|Texas Instruments Incorporated
|8 Channel, SPI, Voltage-Output DAC With Precision Internal Reference
[IBIS Ver]   4.1
[File name]   dacx0508.ibs
[File Rev]   4.0
[Date]   06/21/2018
[Source]
| Texas Instruments Incorporated.
| 12500 TI Blvd
| Dallas, TX -75243
[Notes]   Revision History:
| Rev 4.1: 08/20/2021
| - Added SDO pin Hi-Z mode option version for DAC80508
| Rev 4.0: 06/21/2018
| - Added CLR version for DAC60508 and DAC80508
| Rev 3.0: 05/10/2018
| - Added model for 3.3V operation.
| - Updated C_comp values
| - Model generated from simulations in SPECTRE
| Rev 2.0: 01/17/2018
| - Added YZF package
| Rev 1.0: 01/27/2017
| - Initial version of the model
| - Model generated from simulations in TISPICE
| - C_comp although listed in numerical order of value are
|   obtained from varying PVT conditions. For PVT conditions for
|   each specific value refer the buffer description under
|   respective [Model]. IBIS model user is responsible for using
|   appropriate C_comp to simulate for Signal Integrity.
| - Warnings regarding combined Non-monotonicity of various models have been
|   reviewd and considered minor and can be ignored.
| - Model names with a trailing _1p8 contain the model for
|   1.8V operation. Model names with a trailing _3p0 contain the model
|   for 3.0V operation.Model names with a trailing _3p3 contain the model
|   for 3.3V operation.Model names with a trailing _5p0 contain the model
|   for 5.0V operation.
[Disclaimer]
| This model is designed as an aid for customers of Texas Instruments.
| TI and its licensors and suppliers make no warranties, either expressed
| or implied, with respect to this  model, including the warranties of
| merchantability or fitness for a particular purpose. The model is
| provided solely on an "as is" basis. The entire risk as to its quality
| and performance is with the customer.
| This model is subject to change without notice. Texas Instruments
| Incorporated is not responsible for updating this model.
[Copyright]
 (C) Copyright 2018 Texas Instruments Incorporated.All rights reserved.
| Component DAC60508MRTE
| 16 pin WQFN
| Part # DAC60508MRTE
[Component]   DAC60508MRTE
[Manufacturer]  TI
[Package]   |16 pin WQFN
| variable   typ   min   max
R_pkg   0.1   0.08   0.12
L_pkg   1.0nH   0.8nH   1.2nH
C_pkg   0.2pF   0.16pF   0.24pF
[Pin]  signal_name   model_name   R_pin   L_pin   C_pin
1   REF   NC   NA   NA   NA
2   OUT0   NC   NA   NA   NA
3   OUT1   NC   NA   NA   NA
4   OUT2   NC   NA   NA   NA
5   OUT3   NC   NA   NA   NA
6   GND   GND   NA   NA   NA
7   VDD   POWER   NA   NA   NA
8   OUT4   NC   NA   NA   NA
9   OUT5   NC   NA   NA   NA
10   OUT6   NC   NA   NA   NA
11   OUT7   NC   NA   NA   NA
12   CSB   SDI   NA   NA   NA
13   SCLK   SDI   NA   NA   NA
14   SDI   SDI   NA   NA   NA
15   SDO/ALARMB   SDO   NA   NA   NA
16   VIO   POWER   NA   NA   NA
| Component DAC60508MYZF
| 16 pin WCSP (DSBGA)
| Part # DAC60508MYZF
[Component]   DAC60508MYZF
[Manufacturer]  TI
[Package]   |16 pin WCSP (DSBGA)
|   typ   min   max
R_pkg   0.05541   0.02966   0.07361
L_pkg   0.80718nH   0.45716nH   1.06868nH
C_pkg   0.099388pF   0.08474pF   0.14929pF
[Pin]  signal_name   model_name   R_pin   L_pin   C_pin
C1   REF   NC   NA   NA   NA
C2   OUT0   NC   NA   NA   NA
B1   OUT1   NC   NA   NA   NA
B2   OUT2   NC   NA   NA   NA
A1   OUT3   NC   NA   NA   NA
A2   GND   GND   NA   NA   NA
A3   VDD   POWER   NA   NA   NA
A4   OUT4   NC   NA   NA   NA
B4   OUT5   NC   NA   NA   NA
B3   OUT6   NC   NA   NA   NA
C3   OUT7   NC   NA   NA   NA
C4   CSB   SDI   NA   NA   NA
D4   SCLK   SDI   NA   NA   NA
D3   SDI   SDI   NA   NA   NA
D2   SDO/ALARMB   SDO   NA   NA   NA
D1   VIO   POWER   NA   NA   NA
| Component DAC60508ZRTE
| 16 pin WQFN
| Part # DAC60508ZRTE
[Component]   DAC60508ZRTE
[Manufacturer]  TI
[Package]   |16 pin WQFN
| variable   typ   min   max
R_pkg   0.1   0.08   0.12
L_pkg   1.0nH   0.8nH   1.2nH
C_pkg   0.2pF   0.16pF   0.24pF
[Pin]  signal_name   model_name   R_pin   L_pin   C_pin
1   REF   NC   NA   NA   NA
2   OUT0   NC   NA   NA   NA
3   OUT1   NC   NA   NA   NA
4   OUT2   NC   NA   NA   NA
5   OUT3   NC   NA   NA   NA
6   GND   GND   NA   NA   NA
7   VDD   POWER   NA   NA   NA
8   OUT4   NC   NA   NA   NA
9   OUT5   NC   NA   NA   NA
10   OUT6   NC   NA   NA   NA
11   OUT7   NC   NA   NA   NA
12   CSB   SDI   NA   NA   NA
13   SCLK   SDI   NA   NA   NA
14   SDI   SDI   NA   NA   NA
15   SDO/ALARMB   SDO   NA   NA   NA
16   VIO   POWER   NA   NA   NA
| Component DAC60508ZYZF
| 16 pin WCSP (DSBGA)
| Part # DAC60508ZYZF
[Component]   DAC60508ZYZF
[Manufacturer]  TI
[Package]   |16 pin WCSP (DSBGA)
|   typ   min   max
R_pkg   0.05541   0.02966   0.07361
L_pkg   0.80718nH   0.45716nH   1.06868nH
C_pkg   0.099388pF   0.08474pF   0.14929pF
[Pin]  signal_name   model_name   R_pin   L_pin   C_pin
C1   REF   NC   NA   NA   NA
C2   OUT0   NC   NA   NA   NA
B1   OUT1   NC   NA   NA   NA
B2   OUT2   NC   NA   NA   NA
A1   OUT3   NC   NA   NA   NA
A2   GND   GND   NA   NA   NA
A3   VDD   POWER   NA   NA   NA
A4   OUT4   NC   NA   NA   NA
B4   OUT5   NC   NA   NA   NA
B3   OUT6   NC   NA   NA   NA
C3   OUT7   NC   NA   NA   NA
C4   CSB   SDI   NA   NA   NA
D4   SCLK   SDI   NA   NA   NA
D3   SDI   SDI   NA   NA   NA
D2   SDO/ALARMB   SDO   NA   NA   NA
D1   VIO   POWER   NA   NA   NA
| Component DAC60508MCRTE
| 16 pin WQFN
| Part # DAC60508MCRTE
[Component]   DAC60508MCRTE
[Manufacturer]  TI
[Package]   |16 pin WQFN
| variable   typ   min   max
R_pkg   0.1   0.08   0.12
L_pkg   1.0nH   0.8nH   1.2nH
C_pkg   0.2pF   0.16pF   0.24pF
[Pin]  signal_name   model_name   R_pin   L_pin   C_pin
1   REF   NC   NA   NA   NA
2   OUT0   NC   NA   NA   NA
3   OUT1   NC   NA   NA   NA
4   OUT2   NC   NA   NA   NA
5   OUT3   NC   NA   NA   NA
6   GND   GND   NA   NA   NA
7   VDD   POWER   NA   NA   NA
8   OUT4   NC   NA   NA   NA
9   OUT5   NC   NA   NA   NA
10   OUT6   NC   NA   NA   NA
11   OUT7   NC   NA   NA   NA
12   CSB   SDI   NA   NA   NA
13   SCLK   SDI   NA   NA   NA
14   SDI   SDI   NA   NA   NA
15   CLRB   SDI   NA   NA   NA
16   VIO   POWER   NA   NA   NA
| Component DAC60508MCYZF
| 16 pin WCSP (DSBGA)
| Part # DAC60508MCYZF
[Component]   DAC60508MCYZF
[Manufacturer]  TI
[Package]   |16 pin WCSP (DSBGA)
|   typ   min   max
R_pkg   0.05541   0.02966   0.07361
L_pkg   0.80718nH   0.45716nH   1.06868nH
C_pkg   0.099388pF   0.08474pF   0.14929pF
[Pin]  signal_name   model_name   R_pin   L_pin   C_pin
C1   REF   NC   NA   NA   NA
C2   OUT0   NC   NA   NA   NA
B1   OUT1   NC   NA   NA   NA
B2   OUT2   NC   NA   NA   NA
A1   OUT3   NC   NA   NA   NA
A2   GND   GND   NA   NA   NA
A3   VDD   POWER   NA   NA   NA
A4   OUT4   NC   NA   NA   NA
B4   OUT5   NC   NA   NA   NA
B3   OUT6   NC   NA   NA   NA
C3   OUT7   NC   NA   NA   NA
C4   CSB   SDI   NA   NA   NA
D4   SCLK   SDI   NA   NA   NA
D3   SDI   SDI   NA   NA   NA
D2   CLRB   SDI   NA   NA   NA
D1   VIO   POWER   NA   NA   NA
| Component DAC60508ZCRTE
| 16 pin WQFN
| Part # DAC60508ZCRTE
[Component]   DAC60508ZCRTE
[Manufacturer]  TI
[Package]   |16 pin WQFN
| variable   typ   min   max
R_pkg   0.1   0.08   0.12
L_pkg   1.0nH   0.8nH   1.2nH
C_pkg   0.2pF   0.16pF   0.24pF
[Pin]  signal_name   model_name   R_pin   L_pin   C_pin
1   REF   NC   NA   NA   NA
2   OUT0   NC   NA   NA   NA
3   OUT1   NC   NA   NA   NA
4   OUT2   NC   NA   NA   NA
5   OUT3   NC   NA   NA   NA
6   GND   GND   NA   NA   NA
7   VDD   POWER   NA   NA   NA
8   OUT4   NC   NA   NA   NA
9   OUT5   NC   NA   NA   NA
10   OUT6   NC   NA   NA   NA
11   OUT7   NC   NA   NA   NA
12   CSB   SDI   NA   NA   NA
13   SCLK   SDI   NA   NA   NA
14   SDI   SDI   NA   NA   NA
15   CLRB   SDI   NA   NA   NA
16   VIO   POWER   NA   NA   NA
| Component DAC60508ZCYZF
| 16 pin WCSP (DSBGA)
| Part # DAC60508ZCYZF
[Component]   DAC60508ZCYZF
[Manufacturer]  TI
[Package]   |16 pin WCSP (DSBGA)
|   typ   min   max
R_pkg   0.05541   0.02966   0.07361
L_pkg   0.80718nH   0.45716nH   1.06868nH
C_pkg   0.099388pF   0.08474pF   0.14929pF
[Pin]  signal_name   model_name   R_pin   L_pin   C_pin
C1   REF   NC   NA   NA   NA
C2   OUT0   NC   NA   NA   NA
B1   OUT1   NC   NA   NA   NA
B2   OUT2   NC   NA   NA   NA
A1   OUT3   NC   NA   NA   NA
A2   GND   GND   NA   NA   NA
A3   VDD   POWER   NA   NA   NA
A4   OUT4   NC   NA   NA   NA
B4   OUT5   NC   NA   NA   NA
B3   OUT6   NC   NA   NA   NA
C3   OUT7   NC   NA   NA   NA
C4   CSB   SDI   NA   NA   NA
D4   SCLK   SDI   NA   NA   NA
D3   SDI   SDI   NA   NA   NA
D2   CLRB   SDI   NA   NA   NA
D1   VIO   POWER   NA   NA   NA
| Component DAC70508MRTE
| 16 pin WQFN
| Part # DAC70508MRTE
[Component]   DAC70508MRTE
[Manufacturer]  TI
[Package]   |16 pin WQFN
| variable   typ   min   max
R_pkg   0.1   0.08   0.12
L_pkg   1.0nH   0.8nH   1.2nH
C_pkg   0.2pF   0.16pF   0.24pF
[Pin]  signal_name   model_name   R_pin   L_pin   C_pin
1   REF   NC   NA   NA   NA
2   OUT0   NC   NA   NA   NA
3   OUT1   NC   NA   NA   NA
4   OUT2   NC   NA   NA   NA
5   OUT3   NC   NA   NA   NA
6   GND   GND   NA   NA   NA
7   VDD   POWER   NA   NA   NA
8   OUT4   NC   NA   NA   NA
9   OUT5   NC   NA   NA   NA
10   OUT6   NC   NA   NA   NA
11   OUT7   NC   NA   NA   NA
12   CSB   SDI   NA   NA   NA
13   SCLK   SDI   NA   NA   NA
14   SDI   SDI   NA   NA   NA
15   SDO/ALARMB   SDO   NA   NA   NA
16   VIO   POWER   NA   NA   NA
| Component DAC70508MYZF
| 16 pin WCSP (DSBGA)
| Part # DAC70508MYZF
[Component]   DAC70508MYZF
[Manufacturer]  TI
[Package]   |16 pin WCSP (DSBGA)
|   typ   min   max
R_pkg   0.05541   0.02966   0.07361
L_pkg   0.80718nH   0.45716nH   1.06868nH
C_pkg   0.099388pF   0.08474pF   0.14929pF
[Pin]  signal_name   model_name   R_pin   L_pin   C_pin
C1   REF   NC   NA   NA   NA
C2   OUT0   NC   NA   NA   NA
B1   OUT1   NC   NA   NA   NA
B2   OUT2   NC   NA   NA   NA
A1   OUT3   NC   NA   NA   NA
A2   GND   GND   NA   NA   NA
A3   VDD   POWER   NA   NA   NA
A4   OUT4   NC   NA   NA   NA
B4   OUT5   NC   NA   NA   NA
B3   OUT6   NC   NA   NA   NA
C3   OUT7   NC   NA   NA   NA
C4   CSB   SDI   NA   NA   NA
D4   SCLK   SDI   NA   NA   NA
D3   SDI   SDI   NA   NA   NA
D2   SDO/ALARMB   SDO   NA   NA   NA
D1   VIO   POWER   NA   NA   NA
| Component DAC70508ZRTE
| 16 pin WQFN
| Part # DAC70508ZRTE
[Component]   DAC70508ZRTE
[Manufacturer]  TI
[Package]   |16 pin WQFN
| variable   typ   min   max
R_pkg   0.1   0.08   0.12
L_pkg   1.0nH   0.8nH   1.2nH
C_pkg   0.2pF   0.16pF   0.24pF
[Pin]  signal_name   model_name   R_pin   L_pin   C_pin
1   REF   NC   NA   NA   NA
2   OUT0   NC   NA   NA   NA
3   OUT1   NC   NA   NA   NA
4   OUT2   NC   NA   NA   NA
5   OUT3   NC   NA   NA   NA
6   GND   GND   NA   NA   NA
7   VDD   POWER   NA   NA   NA
8   OUT4   NC   NA   NA   NA
9   OUT5   NC   NA   NA   NA
10   OUT6   NC   NA   NA   NA
11   OUT7   NC   NA   NA   NA
12   CSB   SDI   NA   NA   NA
13   SCLK   SDI   NA   NA   NA
14   SDI   SDI   NA   NA   NA
15   SDO/ALARMB   SDO   NA   NA   NA
16   VIO   POWER   NA   NA   NA
| Component DAC70508ZYZF
| 16 pin WCSP (DSBGA)
| Part # DAC70508ZYZF
[Component]   DAC70508ZYZF
[Manufacturer]  TI
[Package]   |16 pin WCSP (DSBGA)
|   typ   min   max
R_pkg   0.05541   0.02966   0.07361
L_pkg   0.80718nH   0.45716nH   1.06868nH
C_pkg   0.099388pF   0.08474pF   0.14929pF
[Pin]  signal_name   model_name   R_pin   L_pin   C_pin
C1   REF   NC   NA   NA   NA
C2   OUT0   NC   NA   NA   NA
B1   OUT1   NC   NA   NA   NA
B2   OUT2   NC   NA   NA   NA
A1   OUT3   NC   NA   NA   NA
A2   GND   GND   NA   NA   NA
A3   VDD   POWER   NA   NA   NA
A4   OUT4   NC   NA   NA   NA
B4   OUT5   NC   NA   NA   NA
B3   OUT6   NC   NA   NA   NA
C3   OUT7   NC   NA   NA   NA
C4   CSB   SDI   NA   NA   NA
D4   SCLK   SDI   NA   NA   NA
D3   SDI   SDI   NA   NA   NA
D2   SDO/ALARMB   SDO   NA   NA   NA
D1   VIO   POWER   NA   NA   NA
| Component DAC80508MRTE
| 16 pin WQFN
| Part # DAC80508MRTE
[Component]   DAC80508MRTE
[Manufacturer]  TI
[Package]   |16 pin WQFN
| variable   typ   min   max
R_pkg   0.1   0.08   0.12
L_pkg   1.0nH   0.8nH   1.2nH
C_pkg   0.2pF   0.16pF   0.24pF
[Pin]  signal_name   model_name   R_pin   L_pin   C_pin
1   REF   NC   NA   NA   NA
2   OUT0   NC   NA   NA   NA
3   OUT1   NC   NA   NA   NA
4   OUT2   NC   NA   NA   NA
5   OUT3   NC   NA   NA   NA
6   GND   GND   NA   NA   NA
7   VDD   POWER   NA   NA   NA
8   OUT4   NC   NA   NA   NA
9   OUT5   NC   NA   NA   NA
10   OUT6   NC   NA   NA   NA
11   OUT7   NC   NA   NA   NA
12   CSB   SDI   NA   NA   NA
13   SCLK   SDI   NA   NA   NA
14   SDI   SDI   NA   NA   NA
15   SDO/ALARMB   SDO   NA   NA   NA
16   VIO   POWER   NA   NA   NA
| Component DAC80508MRTE_SDOHiZ
| 16 pin WQFN
| Part # DAC80508MRTE
[Component]   DAC80508MRTE_SDOHiZ
[Manufacturer]  TI
[Package]   |16 pin WQFN
| variable   typ   min   max
R_pkg   0.1   0.08   0.12
L_pkg   1.0nH   0.8nH   1.2nH
C_pkg   0.2pF   0.16pF   0.24pF
[Pin]  signal_name   model_name   R_pin   L_pin   C_pin
1   REF   NC   NA   NA   NA
2   OUT0   NC   NA   NA   NA
3   OUT1   NC   NA   NA   NA
4   OUT2   NC   NA   NA   NA
5   OUT3   NC   NA   NA   NA
6   GND   GND   NA   NA   NA
7   VDD   POWER   NA   NA   NA
8   OUT4   NC   NA   NA   NA
9   OUT5   NC   NA   NA   NA
10   OUT6   NC   NA   NA   NA
11   OUT7   NC   NA   NA   NA
12   CSB   SDI   NA   NA   NA
13   SCLK   SDI   NA   NA   NA
14   SDI   SDI   NA   NA   NA
15   SDO/ALARMB   SDI   NA   NA   NA
16   VIO   POWER   NA   NA   NA
| Component DAC80508MYZF
| 16 pin WCSP (DSBGA)
| Part # DAC80508MYZF
[Component]   DAC80508MYZF
[Manufacturer]  TI
[Package]   |16 pin WCSP (DSBGA)
|   typ   min   max
R_pkg   0.05541   0.02966   0.07361
L_pkg   0.80718nH   0.45716nH   1.06868nH
C_pkg   0.099388pF   0.08474pF   0.14929pF
[Pin]  signal_name   model_name   R_pin   L_pin   C_pin
C1   REF   NC   NA   NA   NA
C2   OUT0   NC   NA   NA   NA
B1   OUT1   NC   NA   NA   NA
B2   OUT2   NC   NA   NA   NA
A1   OUT3   NC   NA   NA   NA
A2   GND   GND   NA   NA   NA
A3   VDD   POWER   NA   NA   NA
A4   OUT4   NC   NA   NA   NA
B4   OUT5   NC   NA   NA   NA
B3   OUT6   NC   NA   NA   NA
C3   OUT7   NC   NA   NA   NA
C4   CSB   SDI   NA   NA   NA
D4   SCLK   SDI   NA   NA   NA
D3   SDI   SDI   NA   NA   NA
D2   SDO/ALARMB   SDO   NA   NA   NA
D1   VIO   POWER   NA   NA   NA
| Component DAC80508MYZF_SDOHiZ
| 16 pin WCSP (DSBGA)
| Part # DAC80508MYZF
[Component]   DAC80508MYZF_SDOHiZ
[Manufacturer]  TI
[Package]   |16 pin WCSP (DSBGA)
|   typ   min   max
R_pkg   0.05541   0.02966   0.07361
L_pkg   0.80718nH   0.45716nH   1.06868nH
C_pkg   0.099388pF   0.08474pF   0.14929pF
[Pin]  signal_name   model_name   R_pin   L_pin   C_pin
C1   REF   NC   NA   NA   NA
C2   OUT0   NC   NA   NA   NA
B1   OUT1   NC   NA   NA   NA
B2   OUT2   NC   NA   NA   NA
A1   OUT3   NC   NA   NA   NA
A2   GND   GND   NA   NA   NA
A3   VDD   POWER   NA   NA   NA
A4   OUT4   NC   NA   NA   NA
B4   OUT5   NC   NA   NA   NA
B3   OUT6   NC   NA   NA   NA
C3   OUT7   NC   NA   NA   NA
C4   CSB   SDI   NA   NA   NA
D4   SCLK   SDI   NA   NA   NA
D3   SDI   SDI   NA   NA   NA
D2   SDO/ALARMB   SDI   NA   NA   NA
D1   VIO   POWER   NA   NA   NA
| Component DAC80508ZRTE
| 16 pin WQFN
| Part # DAC80508ZRTE
[Component]   DAC80508ZRTE
[Manufacturer]  TI
[Package]   |16 pin WQFN
| variable   typ   min   max
R_pkg   0.1   0.08   0.12
L_pkg   1.0nH   0.8nH   1.2nH
C_pkg   0.2pF   0.16pF   0.24pF
[Pin]  signal_name   model_name   R_pin   L_pin   C_pin
1   REF   NC   NA   NA   NA
2   OUT0   NC   NA   NA   NA
3   OUT1   NC   NA   NA   NA
4   OUT2   NC   NA   NA   NA
5   OUT3   NC   NA   NA   NA
6   GND   GND   NA   NA   NA
7   VDD   POWER   NA   NA   NA
8   OUT4   NC   NA   NA   NA
9   OUT5   NC   NA   NA   NA
10   OUT6   NC   NA   NA   NA
11   OUT7   NC   NA   NA   NA
12   CSB   SDI   NA   NA   NA
13   SCLK   SDI   NA   NA   NA
14   SDI   SDI   NA   NA   NA
15   SDO/ALARMB   SDO   NA   NA   NA
16   VIO   POWER   NA   NA   NA
| Component DAC80508ZRTE_SDOHiZ
| 16 pin WQFN
| Part # DAC80508ZRTE
[Component]   DAC80508ZRTE_SDOHiZ
[Manufacturer]  TI
[Package]   |16 pin WQFN
| variable   typ   min   max
R_pkg   0.1   0.08   0.12
L_pkg   1.0nH   0.8nH   1.2nH
C_pkg   0.2pF   0.16pF   0.24pF
[Pin]  signal_name   model_name   R_pin   L_pin   C_pin
1   REF   NC   NA   NA   NA
2   OUT0   NC   NA   NA   NA
3   OUT1   NC   NA   NA   NA
4   OUT2   NC   NA   NA   NA
5   OUT3   NC   NA   NA   NA
6   GND   GND   NA   NA   NA
7   VDD   POWER   NA   NA   NA
8   OUT4   NC   NA   NA   NA
9   OUT5   NC   NA   NA   NA
10   OUT6   NC   NA   NA   NA
11   OUT7   NC   NA   NA   NA
12   CSB   SDI   NA   NA   NA
13   SCLK   SDI   NA   NA   NA
14   SDI   SDI   NA   NA   NA
15   SDO/ALARMB   SDI   NA   NA   NA
16   VIO   POWER   NA   NA   NA
| Component DAC80508ZYZF
| 16 pin WCSP (DSBGA)
| Part # DAC80508ZYZF
[Component]   DAC80508ZYZF
[Manufacturer]  TI
[Package]   |16 pin WCSP (DSBGA)
|   typ   min   max
R_pkg   0.05541   0.02966   0.07361
L_pkg   0.80718nH   0.45716nH   1.06868nH
C_pkg   0.099388pF   0.08474pF   0.14929pF
[Pin]  signal_name   model_name   R_pin   L_pin   C_pin
C1   REF   NC   NA   NA   NA
C2   OUT0   NC   NA   NA   NA
B1   OUT1   NC   NA   NA   NA
B2   OUT2   NC   NA   NA   NA
A1   OUT3   NC   NA   NA   NA
A2   GND   GND   NA   NA   NA
A3   VDD   POWER   NA   NA   NA
A4   OUT4   NC   NA   NA   NA
B4   OUT5   NC   NA   NA   NA
B3   OUT6   NC   NA   NA   NA
C3   OUT7   NC   NA   NA   NA
C4   CSB   SDI   NA   NA   NA
D4   SCLK   SDI   NA   NA   NA
D3   SDI   SDI   NA   NA   NA
D2   SDO/ALARMB   SDO   NA   NA   NA
D1   VIO   POWER   NA   NA   NA
| Component DAC80508ZYZF_SDOHiZ
| 16 pin WCSP (DSBGA)
| Part # DAC80508ZYZF
[Component]   DAC80508ZYZF_SDOHiZ
[Manufacturer]  TI
[Package]   |16 pin WCSP (DSBGA)
|   typ   min   max
R_pkg   0.05541   0.02966   0.07361
L_pkg   0.80718nH   0.45716nH   1.06868nH
C_pkg   0.099388pF   0.08474pF   0.14929pF
[Pin]  signal_name   model_name   R_pin   L_pin   C_pin
C1   REF   NC   NA   NA   NA
C2   OUT0   NC   NA   NA   NA
B1   OUT1   NC   NA   NA   NA
B2   OUT2   NC   NA   NA   NA
A1   OUT3   NC   NA   NA   NA
A2   GND   GND   NA   NA   NA
A3   VDD   POWER   NA   NA   NA
A4   OUT4   NC   NA   NA   NA
B4   OUT5   NC   NA   NA   NA
B3   OUT6   NC   NA   NA   NA
C3   OUT7   NC   NA   NA   NA
C4   CSB   SDI   NA   NA   NA
D4   SCLK   SDI   NA   NA   NA
D3   SDI   SDI   NA   NA   NA
D2   SDO/ALARMB   SDI   NA   NA   NA
D1   VIO   POWER   NA   NA   NA
| Component DAC80508MCRTE
| 16 pin WQFN
| Part # DAC80508MCRTE
[Component]   DAC80508MCRTE
[Manufacturer]  TI
[Package]   |16 pin WQFN
| variable   typ   min   max
R_pkg   0.1   0.08   0.12
L_pkg   1.0nH   0.8nH   1.2nH
C_pkg   0.2pF   0.16pF   0.24pF
[Pin]  signal_name   model_name   R_pin   L_pin   C_pin
1   REF   NC   NA   NA   NA
2   OUT0   NC   NA   NA   NA
3   OUT1   NC   NA   NA   NA
4   OUT2   NC   NA   NA   NA
5   OUT3   NC   NA   NA   NA
6   GND   GND   NA   NA   NA
7   VDD   POWER   NA   NA   NA
8   OUT4   NC   NA   NA   NA
9   OUT5   NC   NA   NA   NA
10   OUT6   NC   NA   NA   NA
11   OUT7   NC   NA   NA   NA
12   CSB   SDI   NA   NA   NA
13   SCLK   SDI   NA   NA   NA
14   SDI   SDI   NA   NA   NA
15   CLRB   SDI   NA   NA   NA
16   VIO   POWER   NA   NA   NA
| Component DAC80508MCYZF
| 16 pin WCSP (DSBGA)
| Part # DAC80508MCYZF
[Component]   DAC80508MCYZF
[Manufacturer]  TI
[Package]   |16 pin WCSP (DSBGA)
|   typ   min   max
R_pkg   0.05541   0.02966   0.07361
L_pkg   0.80718nH   0.45716nH   1.06868nH
C_pkg   0.099388pF   0.08474pF   0.14929pF
[Pin]  signal_name   model_name   R_pin   L_pin   C_pin
C1   REF   NC   NA   NA   NA
C2   OUT0   NC   NA   NA   NA
B1   OUT1   NC   NA   NA   NA
B2   OUT2   NC   NA   NA   NA
A1   OUT3   NC   NA   NA   NA
A2   GND   GND   NA   NA   NA
A3   VDD   POWER   NA   NA   NA
A4   OUT4   NC   NA   NA   NA
B4   OUT5   NC   NA   NA   NA
B3   OUT6   NC   NA   NA   NA
C3   OUT7   NC   NA   NA   NA
C4   CSB   SDI   NA   NA   NA
D4   SCLK   SDI   NA   NA   NA
D3   SDI   SDI   NA   NA   NA
D2   CLRB   SDI   NA   NA   NA
D1   VIO   POWER   NA   NA   NA
| Component DAC80508ZCRTE
| 16 pin WQFN
| Part # DAC80508ZCRTE
[Component]   DAC80508ZCRTE
[Manufacturer]  TI
[Package]   |16 pin WQFN
| variable   typ   min   max
R_pkg   0.1   0.08   0.12
L_pkg   1.0nH   0.8nH   1.2nH
C_pkg   0.2pF   0.16pF   0.24pF
[Pin]  signal_name   model_name   R_pin   L_pin   C_pin
1   REF   NC   NA   NA   NA
2   OUT0   NC   NA   NA   NA
3   OUT1   NC   NA   NA   NA
4   OUT2   NC   NA   NA   NA
5   OUT3   NC   NA   NA   NA
6   GND   GND   NA   NA   NA
7   VDD   POWER   NA   NA   NA
8   OUT4   NC   NA   NA   NA
9   OUT5   NC   NA   NA   NA
10   OUT6   NC   NA   NA   NA
11   OUT7   NC   NA   NA   NA
12   CSB   SDI   NA   NA   NA
13   SCLK   SDI   NA   NA   NA
14   SDI   SDI   NA   NA   NA
15   CLRB   SDI   NA   NA   NA
16   VIO   POWER   NA   NA   NA
| Component DAC80508ZCYZF
| 16 pin WCSP (DSBGA)
| Part # DAC80508ZCYZF
[Component]   DAC80508ZCYZF
[Manufacturer]  TI
[Package]   |16 pin WCSP (DSBGA)
|   typ   min   max
R_pkg   0.05541   0.02966   0.07361
L_pkg   0.80718nH   0.45716nH   1.06868nH
C_pkg   0.099388pF   0.08474pF   0.14929pF
[Pin]  signal_name   model_name   R_pin   L_pin   C_pin
C1   REF   NC   NA   NA   NA
C2   OUT0   NC   NA   NA   NA
B1   OUT1   NC   NA   NA   NA
B2   OUT2   NC   NA   NA   NA
A1   OUT3   NC   NA   NA   NA
A2   GND   GND   NA   NA   NA
A3   VDD   POWER   NA   NA   NA
A4   OUT4   NC   NA   NA   NA
B4   OUT5   NC   NA   NA   NA
B3   OUT6   NC   NA   NA   NA
C3   OUT7   NC   NA   NA   NA
C4   CSB   SDI   NA   NA   NA
D4   SCLK   SDI   NA   NA   NA
D3   SDI   SDI   NA   NA   NA
D2   CLRB   SDI   NA   NA   NA
D1   VIO   POWER   NA   NA   NA
|   Model Selectors
[Model Selector]  SDO
SDO_5p0  sdata buffer at 5.0V operation.
SDO_3p0  sdata buffer at 3.0V operation.
SDO_3p3  sdata buffer at 3.3V operation.
SDO_1p8  sdata buffer at 1.8V operation.
[Model Selector]  SDI
SDI_5p0  sdata buffer at 5.0V operation.
SDI_3p0  sdata buffer at 3.0V operation.
SDI_3p3  sdata buffer at 3.3V operation.
SDI_1p8  sdata buffer at 1.8V operation.
| Models and submodels in the file (8): SDO_5p0 (Output), SDO_3p0 (Output), SDO_3p3 (Output), SDO_1p8 (Output), SDI_5p0 (Input), SDI_3p0 (Input), SDI_3p3 (Input), SDI_1p8 (Input)
